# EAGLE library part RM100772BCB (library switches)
Rotary Switch 8 Position SP7T 500mA (DC) 24VDC Through Hole
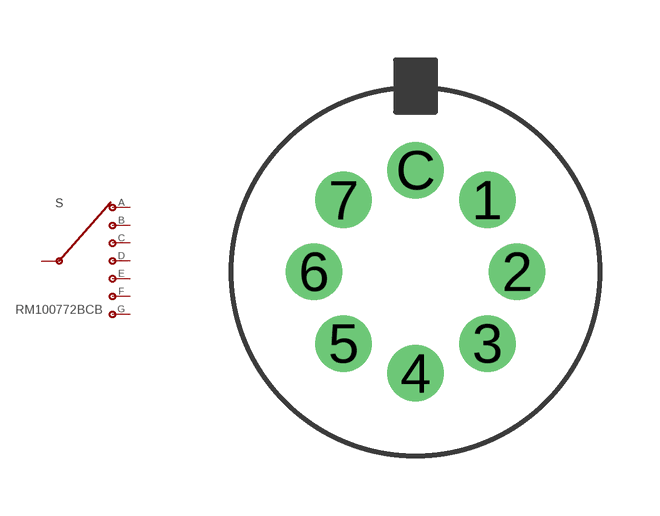
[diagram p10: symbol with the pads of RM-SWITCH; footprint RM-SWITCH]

Designator prefix S

## RM100772BCB  [RM-SWITCH]
1  A
2  B
3  C
4  D
5  E
6  F
7  G
C  INPUT

## Footprint RM-SWITCH (pad centres in mm)
drill 0.9: 1 1.796,1.796; 2 2.54,0; 3 1.796,-1.796; 4 0,-2.54; 5 -1.796,-1.796; 6 -2.54,0; 7 -1.796,1.796; C 0,2.54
